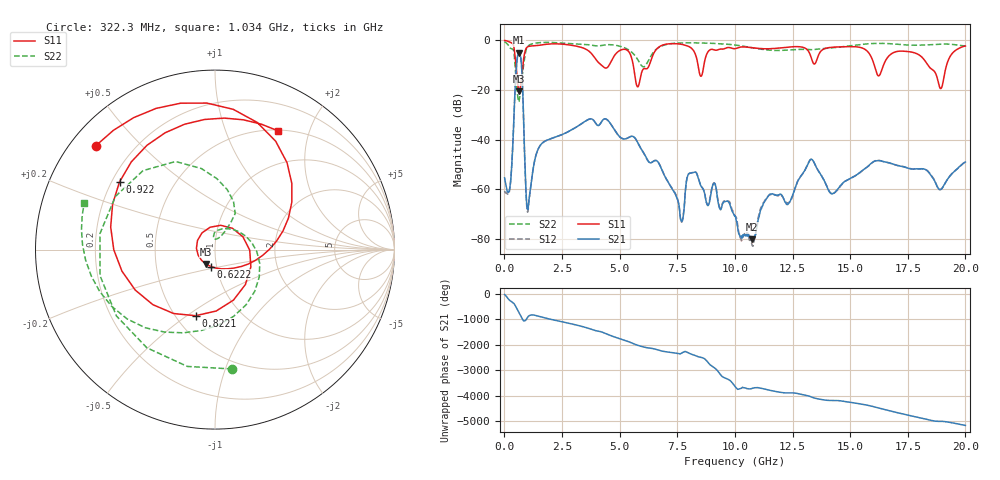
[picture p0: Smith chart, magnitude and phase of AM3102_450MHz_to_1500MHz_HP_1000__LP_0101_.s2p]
!Agilent Technologies,E8364B,MY43040894,A.07.50.67
!Agilent E8364B: A.07.50.67
!Date: Thursday, January 11, 2018 05:57:31
!Correction: S11(Full 2 Port(1,2))
!S21(Full 2 Port(1,2))
!S12(Full 2 Port(1,2))
!S22(Full 2 Port(1,2))
!S2P File: Measurements: S11, S21, S12, S22:
# Hz S  dB  R 50
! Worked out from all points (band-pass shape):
!   1601 points, 10 MHz to 20 GHz, reference 50 ohm
!   highest |S21| = -4.94 dB at 622.2 MHz (marker M1); lowest = -80.1 dB at 10.73 GHz (marker M2)
!   |S21| within 3 dB of the highest: 548.9 MHz to 723.7 MHz (174.7 MHz wide, 27.5 % of centre)
!   lowest |S11| = -20.5 dB at 634.7 MHz (marker M3), VSWR 1.21, Z = 44.7 - j7.27 ohm
!   |S11| at or under -10 dB: 5.59 GHz to 6.287 GHz (696.3 MHz wide, 11.7 % of centre); 16.05 GHz to 16.45 GHz (401.4 MHz wide, 2.47 % of centre); 18.37 GHz to 19.18 GHz (811.8 MHz wide, 4.32 % of centre)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
!   |S22| runs from -24.8 to -0.6 dB; largest |S21 - S12| = 0.0071
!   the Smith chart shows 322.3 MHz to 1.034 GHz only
!   S11 on the Smith chart (normalised r, x): 322.3 MHz: 0.07, +0.37; 622.2 MHz: 0.94, -0.18; 822.1 MHz: 0.62, -0.54; 922 MHz: 0.23, +0.30; 1.034 GHz: 0.51, +1.54
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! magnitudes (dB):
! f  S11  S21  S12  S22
! 10 MHz  -0.1  -55.4  -60.7  -0.6
! 322.3 MHz  -1.1  -50.0  -50.1  -3.5
! 622.2 MHz  -20.3  -4.9  -4.9  -24.8
! 634.7 MHz  -20.5  -5.0  -5.0  -24.6
! 822.1 MHz  -8.3  -27.9  -28.2  -10.7
! 922 MHz  -3.7  -57.3  -58.4  -4.7
! 1.034 GHz  -2.5  -67.4  -68.2  -2.2
! 1.559 GHz  -1.9  -42.3  -42.3  -0.9
! 3.346 GHz  -2.9  -33.6  -33.6  -1.6
! 5.32 GHz  -3.9  -39.5  -39.5  -3.5
! 5.782 GHz  -18.7  -41.1  -41.1  -7.7
! 6.682 GHz  -2.9  -49.2  -49.2  -3.0
! 7.681 GHz  -1.6  -72.9  -73.2  -1.0
! 8.218 GHz  -4.3  -53.2  -53.0  -1.0
! 8.531 GHz  -14.5  -58.7  -58.6  -1.1
! 10.01 GHz  -3.4  -70.6  -70.8  -1.9
! 10.73 GHz  -3.0  -80.1  -81.8  -2.9
! 13.34 GHz  -7.8  -48.0  -48.0  -3.8
! 14.23 GHz  -2.8  -61.8  -61.9  -3.0
! 16.68 GHz  -6.3  -49.3  -49.3  -1.3
! 18.93 GHz  -19.5  -60.1  -60.1  -1.5
! 20 GHz  -2.3  -49.0  -49.0  -2.3
